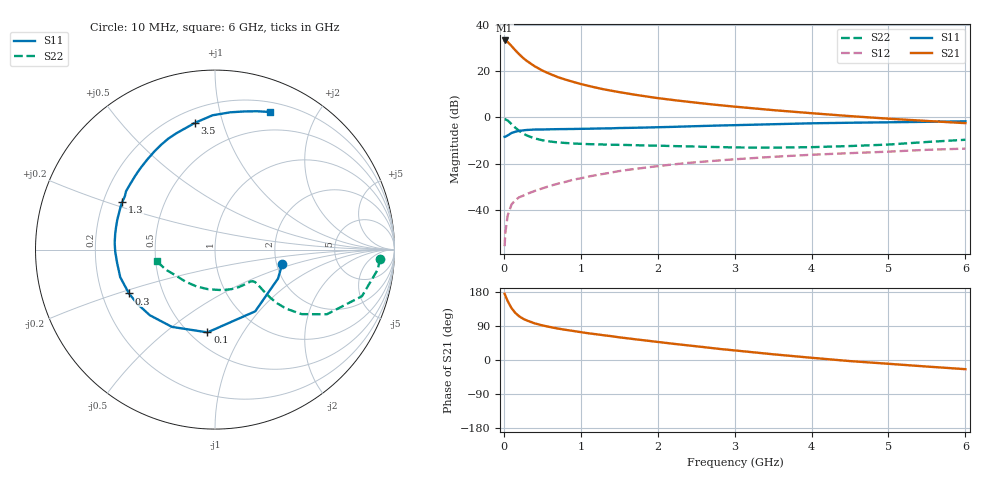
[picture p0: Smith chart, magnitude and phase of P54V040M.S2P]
! SIEMENS Small Signal Semiconductors
! BFP183
! Si NPN RF Bipolar Junction Transistor in SOT143
! VCE = 4 V  IC = 40 mA
! Common Emitter S-Parameters:  March  1996
# GHz  S  MA  R  50
!  f  S11  S21  S12  S22
! GHz  MAG  ANG  MAG  ANG  MAG  ANG  MAG  ANG
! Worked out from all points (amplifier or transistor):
!   36 points, 10 MHz to 6 GHz, reference 50 ohm
!   highest |S21| = 33.1 dB at 10 MHz (marker M1)
!   |S21| within 3 dB of that: start of sweep to 116 MHz
!   unconditionally stable (mu >= 1): 501.3 MHz to 5.783 GHz
!   at 250 MHz: K = 0.69, MSG = 29.7 dB, |S12| = -33.7 dB
!   at 1.4 GHz: K = 1.23, MAG = 14.7 dB, |S12| = -23.7 dB
!   at 6 GHz: K = 0.98, MSG = 5.5 dB, |S12| = -13.4 dB
!   S11 on the Smith chart (normalised r, x): 10 MHz: 2.15, -0.40; 100 MHz: 0.61, -0.71; 300 MHz: 0.32, -0.22; 1.3 GHz: 0.28, +0.22; 3.5 GHz: 0.28, +0.81; 6 GHz: 0.30, +1.43
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0.01  0.3832 -12.1  45.38 174.7  0.0017 77.7  0.9219 -3.2
0.02  0.3864 -24.7  45.05 169.9  0.0034 79.6  0.9127 -7.1
0.05  0.4105 -56.9  42.11 155.4  0.0078 73.6  0.8589 -17.6
0.1  0.4631 -95.2  34.37 136.9  0.0134 59.5  0.7203 -30.0
0.15  0.4929 -119.1  27.82 124.1  0.0167 53.6  0.6017 -36.7
0.2  0.5154 -134.8  22.84 115.3  0.0192 52.4  0.5146 -39.7
0.25  0.5275 -144.9  19.1 108.9  0.0207 50.6  0.4539 -40.9
0.3  0.538 -153.0  16.41 104.2  0.0226 51.6  0.4085 -41.0
0.4  0.5499 -163.7  12.68 96.8  0.0262 54.3  0.3548 -40.4
0.5  0.5504 -172.2  10.22 91.4  0.0298 54.7  0.323 -39.7
0.6  0.556 -178.8  8.647 87.0  0.0336 56.3  0.3037 -39.2
0.7  0.5602 176.2  7.393 83.1  0.0375 58.0  0.2905 -39.0
0.8  0.5625 171.5  6.534 79.7  0.041 58.2  0.2826 -39.3
1.1  0.572 159.4  4.783 70.5  0.0535 59.3  0.2668 -41.6
1.3  0.581 152.9  4.03 65.2  0.0613 58.7  0.2617 -44.5
1.7  0.6002 140.1  3.089 54.9  0.078 56.4  0.2533 -51.4
2.2  0.6277 127.0  2.374 42.9  0.0976 52.2  0.2421 -62.2
2.8  0.6708 112.8  1.84 29.3  0.119 46.4  0.2306 -78.1
3.5  0.715 99.0  1.438 15.1  0.1422 40.0  0.2242 -99.6
4.5  0.7695 83.7  1.069 -2.9  0.1707 30.3  0.2427 -132.7
5.5  0.806 73.0  0.841 -17.3  0.2012 22.1  0.2969 -158.1
6  0.8252 68.3  0.755 -24.2  0.2137 17.2  0.3311 -168.9
